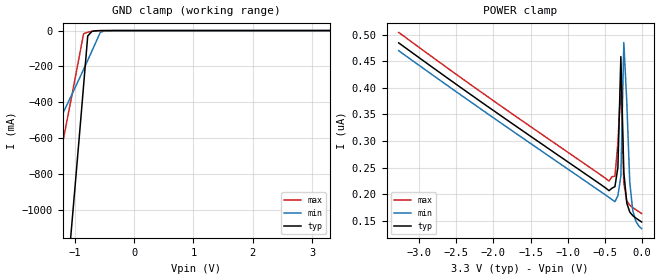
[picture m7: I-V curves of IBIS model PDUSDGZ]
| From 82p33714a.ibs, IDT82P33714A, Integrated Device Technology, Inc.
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|   Model PDUSDGZ
[Model]  PDUSDGZ
Model_type Input
Polarity   Non-Inverting
Vinl =   0.8000V
Vinh =   2.0000V
C_comp   2.6812pF   2.6701pF   2.6826pF
[Temperature Range]   25.0000   0.1250k   -40.0000
[Voltage Range]   3.3000V   3.0000V   3.6000V
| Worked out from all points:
|   GND clamp passes 1 mA (typ) near -0.64 V on its own axis
[GND_clamp]
|Voltage   I(typ)   I(min)   I(max)
-3.3V     -8.473A    -1.702A    -3.669A
-2.25V    -5.322A    -1.129A    -2.26A
-2.18V    -5.094A    -1.087A    -2.158A
-1.55V    -2.941A    -695.3mA   -1.195A
-1.48V    -2.689A    -649.5mA   -1.083A
-1.06V    -1.126A    -365.1mA   -383.4mA
-850mV    -308.3mA   -216.3mA   -17.67mA
-780mV    -30.2mA    -165.7mA   -8.762mA
-710mV    -4.268mA   -114.6mA   -4.618mA
-570mV    -221.6uA   -10.81mA   -478.7uA
-500mV    -88.67uA   -1.744mA   -148.1uA
3.3V      145.9nA    233.6nA    133.9nA
[POWER_clamp]
|Voltage   I(typ)   I(min)   I(max)
-3.28V    484.3nA    469.6nA    504nA
-440mV    206.6nA    193.8nA    224.5nA
-400mV    211.3nA    189.9nA    232.8nA
-360mV    214.2nA    185.9nA    233.8nA
-320mV    250.6nA    197.2nA    296.5nA
-280mV    458.6nA    233.6nA    406nA
-240mV    241nA      484.9nA    220.6nA
-200mV    183.2nA    373.1nA    187.4nA
-160mV    166.5nA    222.6nA    179.2nA
-120mV    159.8nA    169.6nA    174.8nA
-80mV     155.4nA    149.7nA    171nA
0V        147.8nA    135.2nA    163.6nA
